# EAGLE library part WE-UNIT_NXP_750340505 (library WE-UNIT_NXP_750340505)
Off-Line Transformer WE-Unit NXP - Nominal input voltage: 85-265 VAC - Operating temperature: -40°C to +125 °C - Isolation voltage 4 kVAC -- Especially designed for several ICs from NXP SSL2101 -- Universal input -- Smart meters -- Dimmable 12 V LED driver -- Offline-switch mode power supplies
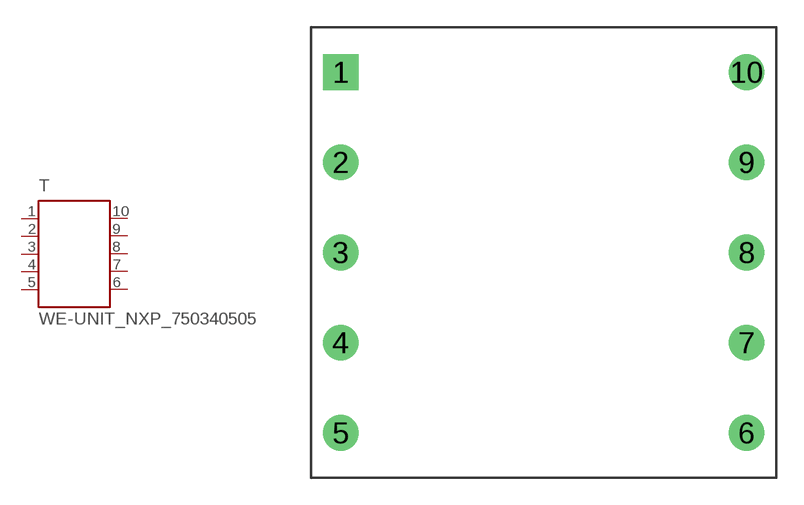
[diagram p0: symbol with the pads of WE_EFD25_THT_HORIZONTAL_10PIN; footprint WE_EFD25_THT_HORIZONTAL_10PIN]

Designator prefix T

## WE-UNIT_NXP_750340505 (MPN: 750340505; OC_FARNELL: 1849059; OC_NEWARK: 13T9834; PACKAGE: EFD25; SUPPLIER: Würth Elektronik eiSos GmbH)  [WE_EFD25_THT_HORIZONTAL_10PIN]
1  1  pas
2  2  pas
3  3  pas
4  4  pas
5  5  pas
6  6  pas
7  7  pas
8  8  pas
9  9  pas
10  10  pas

## Footprint WE_EFD25_THT_HORIZONTAL_10PIN (pad centres in mm)
Transformer, EFD25 THT Horizontal 10Pins
drill 1.32 square: 1 -11.25,10
drill 1.32: 2 -11.25,5; 3 -11.25,0; 4 -11.25,-5; 5 -11.25,-10; 6 11.25,-10; 7 11.25,-5; 8 11.25,0; 9 11.25,5; 10 11.25,10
